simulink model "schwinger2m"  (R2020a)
settings: Solver=ode45  StartTime=0.0  StopTime=40  RelTol=1e-3  EnableMultiTasking=on

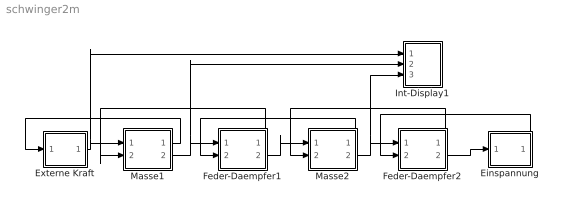
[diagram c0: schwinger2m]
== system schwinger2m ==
  Einspannung : Subsystem  mask(Einspannung){v0=0}
      mask prompts: v0 "Geschwindigkeit"
  Externe Kraft : Subsystem  mask(Externe Kraft, harmonisch){F0=1, omega=3}
      mask prompts: F0 "Kraft-Amplitude [N]"; omega "Kreisfrequenz [1/s]"
  Feder-Daempfer1 : Subsystem  mask(Feder-Daempfer){c=1, b=1, x0=0}
      mask prompts: c "Federsteifigkeit"; b "Daempfung"; x0 "Vorspannungslaenge"
  Feder-Daempfer2 : Subsystem  mask(Feder-Daempfer){c=1, b=1, x0=0}
      mask prompts: c "Federsteifigkeit"; b "Daempfung"; x0 "Vorspannungslaenge"
  Int-Display1 : Subsystem
  Masse1 : Subsystem  mask(Masse){m=1, v0=0}
      mask prompts: m "Masse"; v0 "Anfangsgeschwindigkeit"
  Masse2 : Subsystem  mask(Masse){m=1, v0=0}
      mask prompts: m "Masse"; v0 "Anfangsgeschwindigkeit"
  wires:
  Externe Kraft/1(F) -> Masse1/1(Fl), Int-Display1/1(In1)
  Masse1/1(vl) -> Externe Kraft/1(v)
  Masse1/2(vr) -> Feder-Daempfer1/1(vl), Int-Display1/2(In2)
  Feder-Daempfer1/1(Fl) -> Masse1/2(Fr)
  Feder-Daempfer1/2(Fr) -> Masse2/1(Fl)
  Masse2/1(vl) -> Feder-Daempfer1/2(vr)
  Masse2/2(vr) -> Int-Display1/3(In3), Feder-Daempfer2/1(vl)
  Feder-Daempfer2/1(Fl) -> Masse2/2(Fr)
  Feder-Daempfer2/2(Fr) -> Einspannung/1(F)
  Einspannung/1(v) -> Feder-Daempfer2/2(vr)

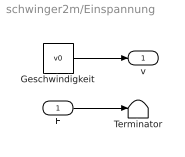
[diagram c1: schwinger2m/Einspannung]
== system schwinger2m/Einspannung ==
  F : Inport
  Geschwindigkeit : Constant  Value=v0
  Terminator : Terminator
  v : Outport
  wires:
  Geschwindigkeit/1 -> v/1
  F/1 -> Terminator/1

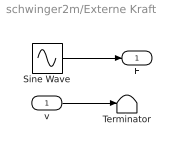
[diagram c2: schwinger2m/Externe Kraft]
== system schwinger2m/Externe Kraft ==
  v : Inport
  Sine Wave : Sin  Amplitude=F0  Frequency=omega  SampleTime=0
  Terminator : Terminator
  F : Outport
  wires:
  Sine Wave/1 -> F/1
  v/1 -> Terminator/1

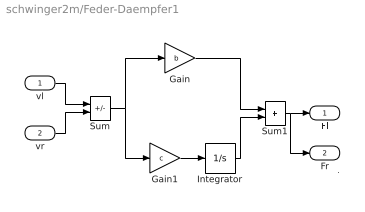
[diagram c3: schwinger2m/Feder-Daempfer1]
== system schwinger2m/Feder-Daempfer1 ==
  note: .
  vl : Inport
  vr : Inport  Port=2
  Gain : Gain  Gain=b  SaturateOnIntegerOverflow=on
  Gain1 : Gain  Gain=c  SaturateOnIntegerOverflow=on
  Integrator : Integrator  InitialCondition=x0/c
  Sum : Sum  Inputs=+-  SaturateOnIntegerOverflow=on
  Sum1 : Sum  SaturateOnIntegerOverflow=on
  Fl : Outport
  Fr : Outport  Port=2
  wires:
  Sum1/1 -> Fl/1, Fr/1
  Gain/1 -> Sum1/1
  Integrator/1 -> Sum1/2
  vl/1 -> Sum/1
  vr/1 -> Sum/2
  Sum/1 -> Gain/1, Gain1/1
  Gain1/1 -> Integrator/1

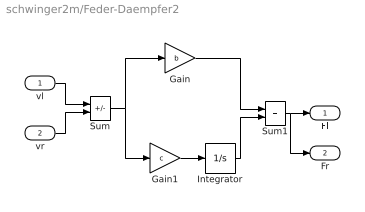
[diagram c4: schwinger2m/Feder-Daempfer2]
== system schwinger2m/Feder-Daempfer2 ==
  vl : Inport
  vr : Inport  Port=2
  Gain : Gain  Gain=b  SaturateOnIntegerOverflow=on
  Gain1 : Gain  Gain=c  SaturateOnIntegerOverflow=on
  Integrator : Integrator  InitialCondition=x0/c
  Sum : Sum  Inputs=+-  SaturateOnIntegerOverflow=on
  Sum1 : Sum  SaturateOnIntegerOverflow=on
  Fl : Outport
  Fr : Outport  Port=2
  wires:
  Gain1/1 -> Integrator/1
  Sum/1 -> Gain1/1, Gain/1
  vr/1 -> Sum/2
  vl/1 -> Sum/1
  Integrator/1 -> Sum1/2
  Gain/1 -> Sum1/1
  Sum1/1 -> Fr/1, Fl/1

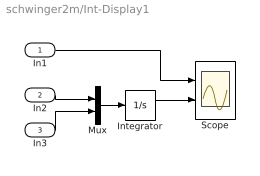
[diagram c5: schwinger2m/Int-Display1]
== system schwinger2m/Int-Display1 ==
  In1 : Inport
  In2 : Inport  Port=2
  In3 : Inport  Port=3
  Integrator : Integrator
  Mux : Mux  Inputs=2
  Scope : Scope  NumInputPorts=2
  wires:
  In3/1 -> Mux/2
  In2/1 -> Mux/1
  Mux/1 -> Integrator/1
  Integrator/1 -> Scope/2
  In1/1 -> Scope/1

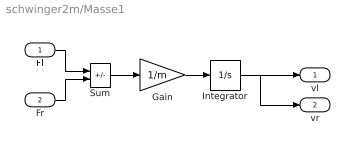
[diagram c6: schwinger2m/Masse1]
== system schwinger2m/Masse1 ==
  note: .
  Fl : Inport
  Fr : Inport  Port=2
  Gain : Gain  Gain=1/m  SaturateOnIntegerOverflow=on
  Integrator : Integrator  InitialCondition=v0
  Sum : Sum  Inputs=+-  SaturateOnIntegerOverflow=on
  vl : Outport
  vr : Outport  Port=2
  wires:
  Integrator/1 -> vl/1, vr/1
  Gain/1 -> Integrator/1
  Sum/1 -> Gain/1
  Fr/1 -> Sum/2
  Fl/1 -> Sum/1

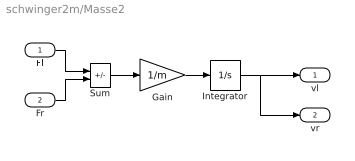
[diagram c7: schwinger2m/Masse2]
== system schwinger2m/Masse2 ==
  Fl : Inport
  Fr : Inport  Port=2
  Gain : Gain  Gain=1/m  SaturateOnIntegerOverflow=on
  Integrator : Integrator  InitialCondition=v0
  Sum : Sum  Inputs=+-  SaturateOnIntegerOverflow=on
  vl : Outport
  vr : Outport  Port=2
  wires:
  Fl/1 -> Sum/1
  Fr/1 -> Sum/2
  Sum/1 -> Gain/1
  Gain/1 -> Integrator/1
  Integrator/1 -> vr/1, vl/1
